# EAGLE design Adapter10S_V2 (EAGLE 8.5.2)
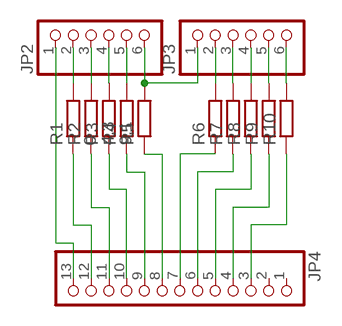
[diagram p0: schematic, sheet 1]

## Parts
JP2  PINHD-1X6  [1X06]
JP3  PINHD-1X6  [1X06]
JP4  PINHD-1X13  [1X13]
R1  0  R-EU_M0805  [M0805]
R2  4,3  R-EU_M0805  [M0805]
R3  9,1  R-EU_M0805  [M0805]
R4  R-EU_M0805  [M0805]
R5  R-EU_M0805  [M0805]
R6  R-EU_M0805  [M0805]
R7  R-EU_M0805  [M0805]
R8  R-EU_M0805  [M0805]
R9  R-EU_M0805  [M0805]
R10  R-EU_M0805  [M0805]

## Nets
GND: JP2.1 JP4.13
N$2: JP2.2 R1.2
N$3: JP2.3 R2.2
N$4: JP2.4 R3.2
N$5: JP2.5 R4.2
N$6: JP2.6 JP3.1 R5.2
N$7: JP3.2 R6.2
N$8: JP3.3 R7.2
N$9: JP3.4 R8.2
N$10: JP3.5 R9.2
N$11: JP3.6 R10.2
N$12: JP4.12 R1.1
N$13: JP4.11 R2.1
N$14: JP4.10 R3.1
N$15: JP4.8 R5.1
N$16: JP4.9 R4.1
N$17: JP4.7 R6.1
N$18: JP4.6 R7.1
N$19: JP4.5 R8.1
N$20: JP4.4 R9.1
N$21: JP4.3 R10.1
Unconnected: JP4.1 JP4.2

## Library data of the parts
JP2 JP3 = pinhead:PINHD-1X6: PIN HEADER
JP4 = pinhead:PINHD-1X13: PIN HEADER
R1-R10 = resistor:R-EU_: RESISTOR, European symbol

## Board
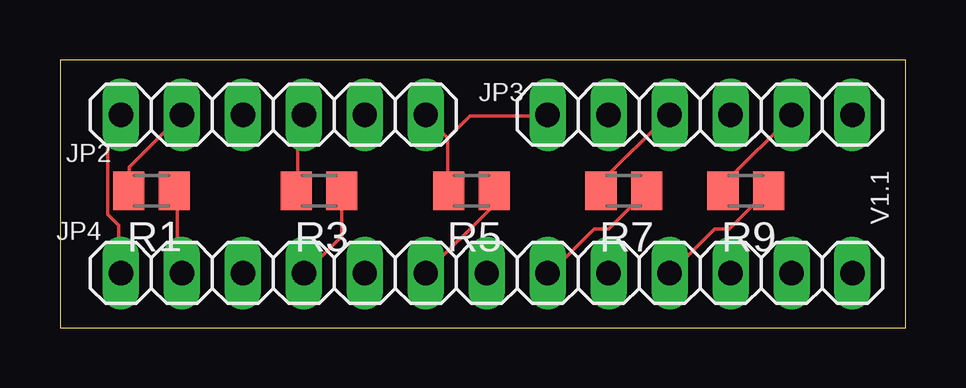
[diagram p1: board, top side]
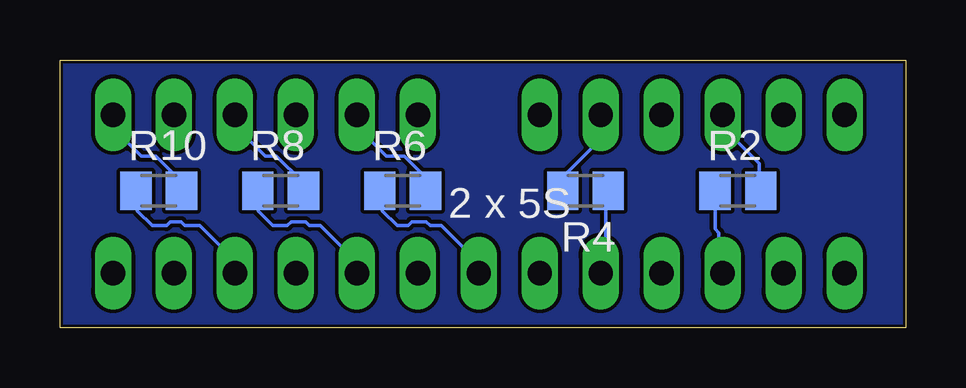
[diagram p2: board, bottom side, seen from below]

Size 35.23 x 11.18 mm. Coordinates in mm from the lower left corner, seen from the top.
Outline: 0,0 35.23,0 35.23,11.18 0,11.18 0,0
Copper layers (1*16): Top 0.035mm / dielectric 1.5mm / Bottom 0.035mm
Design rules "default *": minimum track width 6mil, minimum drill 0.35mm, track to track 6mil, track to pad 6mil, pad to pad 6mil, via to via 6mil, smd to smd 6mil, copper to edge 5mil, drill to drill 6mil, minimum pad ring 10mil, minimum via ring 8mil, stop-mask expansion 4mil, vias tented up to drill 0mil, thermal gap 10mil

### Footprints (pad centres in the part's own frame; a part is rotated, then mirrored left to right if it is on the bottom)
1X06 = drill 1.016 long: 1 -6.35,0; 2 -3.81,0; 3 -1.27,0; 4 1.27,0; 5 3.81,0; 6 6.35,0
1X13 = drill 1.016 long: 1 -15.24,0; 2 -12.7,0; 3 -10.16,0; 4 -7.62,0; 5 -5.08,0; 6 -2.54,0; 7 0,0; 8 2.54,0; 9 5.08,0; 10 7.62,0; 11 10.16,0; 12 12.7,0; 13 15.24,0
M0805 = smd 1.3 x 1.6: 1 -0.95,0; 2 0.95,0

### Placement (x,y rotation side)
JP2  8.89,8.89 0 top
JP3  26.67,8.89 0 top
JP4  17.78,2.29 180 top
R1  3.81,5.71 180 top
R2  6.99,5.71 0 bottom
R3  10.79,5.71 180 top
R4  13.34,5.71 180 bottom
R5  17.14,5.71 180 top
R6  20.95,5.71 0 bottom
R7  23.5,5.71 180 top
R8  26.04,5.71 0 bottom
R9  28.57,5.71 180 top
R10  31.11,5.71 0 bottom

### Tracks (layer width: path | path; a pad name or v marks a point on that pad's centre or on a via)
GND
  Top 0.152: JP4.13 2.44,2.29 2.44,4.27 1.98,4.72 1.98,8.38 2.44,8.84 JP2.1
N$1
  pour Bottom: 0,11.18 35.23,11.18 35.23,0 0,0
N$2
  Top 0.152: JP2.2 2.9,6.71 2.9,5.79 R1.2
N$3
  Bottom 0.152: JP2.3 7.62,8.38 6.1,6.86 6.1,5.79 R2.2
N$4
  Top 0.152: R3.2 9.91,5.79 9.91,8.69 10.06,8.84 JP2.4
N$5
  Bottom 0.152: R4.2 14.17,5.79 14.17,6.4 12.8,7.77 12.8,8.84 JP2.5
N$6
  Top 0.152: 16.15,7.92 16.15,5.79 R5.2 | 16.15,7.92 15.24,8.84 JP2.6 | 16.15,7.92 17.07,8.84 20.27,8.84 JP3.1
N$7
  Bottom 0.152: JP3.2 22.86,8.38 21.64,7.16 20.88,7.16 20.12,6.4 20.12,5.79 R6.2
N$8
  Top 0.152: R7.2 22.55,5.79 22.55,6.1 25.3,8.84 JP3.3
N$9
  Bottom 0.152: R8.2 25.15,5.79 25.15,6.1 26.21,7.16 26.67,7.16 27.89,8.38 27.89,8.84 JP3.4
N$10
  Top 0.152: R9.2 27.74,5.79 27.74,6.1 30.48,8.84 JP3.5
N$11
  Bottom 0.152: R10.2 30.18,5.79 30.18,6.1 31.24,7.16 31.85,7.16 32.92,8.23 32.92,8.84 JP3.6
N$12
  Top 0.152: R1.1 4.88,5.64 4.88,2.44 5.03,2.29 JP4.12
N$13
  Bottom 0.152: JP4.11 7.77,2.44 7.77,3.96 7.92,4.12 7.92,5.64 R2.1
N$14
  Top 0.152: R3.1 11.73,5.64 11.73,3.81 10.21,2.29 JP4.10
N$15
  Top 0.152: JP4.8 17.98,5.03 17.98,5.64 R5.1
N$16
  Bottom 0.152: R4.1 12.5,5.64 12.5,2.44 12.65,2.29 JP4.9
N$17
  Bottom 0.152: R6.1 21.79,5.64 21.79,4.88 21.18,4.27 20.73,4.27 20.57,4.42 19.96,4.42 19.81,4.27 19.36,4.27 17.83,2.74 17.83,2.29 JP4.7
N$18
  Top 0.152: R7.1 24.38,5.64 22.86,4.12 22.25,4.12 20.42,2.29 JP4.6
N$19
  Bottom 0.152: JP4.5 22.86,2.74 24.38,4.27 24.84,4.27 24.99,4.42 25.6,4.42 25.76,4.27 26.36,4.27 26.98,4.88 26.98,5.64 R8.1
N$20
  Top 0.152: R9.1 29.41,5.64 27.89,4.12 27.28,4.12 25.45,2.29 JP4.4
N$21
  Bottom 0.152: R10.1 32,5.64 32,4.88 31.39,4.27 30.79,4.27 30.63,4.42 30.18,4.42 30.02,4.27 29.41,4.27 28.04,2.9 28.04,2.29 JP4.3

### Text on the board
tPlace: V1.1
bNames: 2 x 5S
